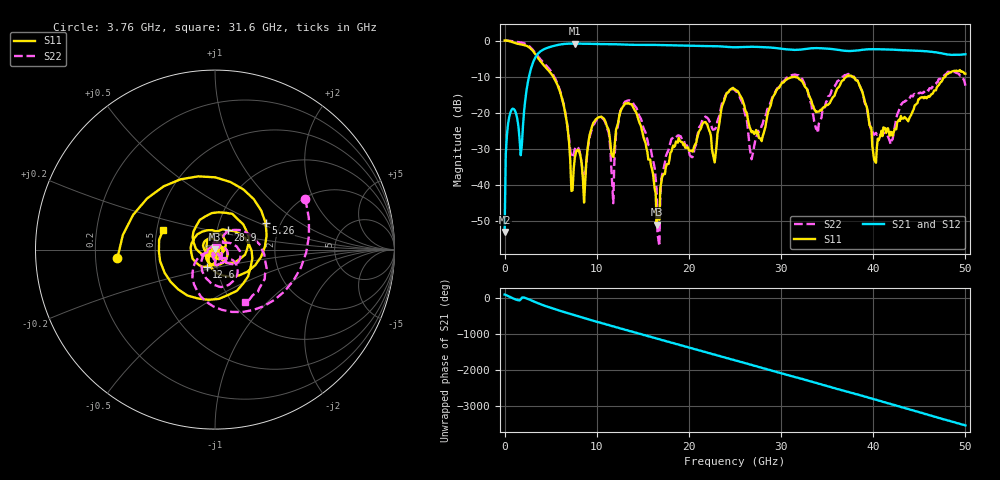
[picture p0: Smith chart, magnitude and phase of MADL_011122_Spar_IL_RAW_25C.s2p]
#	HZ	S	DB	R	50
!Frequency	S11 (dB)	S11-Ang	S21 (dB)	S21-Ang	S12 (dB)	S12-Ang	S22 (dB)	S22-Ang
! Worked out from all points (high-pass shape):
!   401 points, 10 MHz to 50 GHz, reference 50 ohm
!   highest |S21| = -0.85 dB at 7.63 GHz (marker M1); lowest = -53.1 dB at 10 MHz (marker M2)
!   |S21| within 3 dB of the highest: 3.567 GHz to 48 GHz (44.43 GHz wide, 172 % of centre); 49.825 GHz to end of sweep
!   lowest |S11| = -51.0 dB at 16.5 GHz (marker M3), VSWR 1.01, Z = 49.8 + j0.209 ohm
!   |S11| at or under -10 dB: 5.275 GHz to 37.1 GHz (31.83 GHz wide, 150 % of centre); 37.71 GHz to 47.82 GHz (10.1 GHz wide, 23.6 % of centre)
!   |S22| runs from -57.0 to 0.0 dB; largest |S21 - S12| = 0.016
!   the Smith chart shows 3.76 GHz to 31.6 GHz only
!   S11 on the Smith chart (normalised r, x): 3.76 GHz: 0.29, -0.04; 5.26 GHz: 1.67, +0.55; 12.6 GHz: 0.90, -0.17; 28.9 GHz: 1.12, +0.25; 31.6 GHz: 0.54, +0.13
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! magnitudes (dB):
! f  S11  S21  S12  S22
! 10 MHz  0.0  -53.1  -53.8  0.0
! 635 MHz  -0.3  -20.0  -20.0  -0.1
! 1.76 GHz  -1.1  -31.8  -31.7  -0.5
! 3.76 GHz  -5.3  -3.3  -3.3  -4.8
! 5.26 GHz  -9.9  -1.5  -1.5  -9.4
! 7.63 GHz  -32.4  -0.8  -0.8  -30.1
! 8.38 GHz  -34.2  -0.9  -0.9  -34.3
! 10.4 GHz  -21.2  -1.0  -1.0  -21.4
! 11.8 GHz  -32.3  -1.0  -1.0  -45.1
! 12.6 GHz  -19.5  -1.1  -1.1  -19.3
! 14.8 GHz  -23.7  -1.2  -1.2  -21.7
! 16.5 GHz  -51.0  -1.2  -1.2  -41.2
! 16.8 GHz  -49.7  -1.2  -1.2  -57.0
! 18.1 GHz  -30.8  -1.3  -1.3  -27.3
! 25.1 GHz  -13.8  -1.9  -1.8  -14.1
! 26.9 GHz  -25.1  -1.7  -1.7  -31.8
! 28.9 GHz  -17.8  -1.9  -1.9  -16.9
! 31.6 GHz  -10.2  -2.6  -2.6  -9.5
! 33.4 GHz  -17.8  -2.1  -2.1  -19.9
! 37.4 GHz  -9.8  -2.9  -2.9  -9.5
! 41.8 GHz  -26.4  -2.5  -2.5  -27.9
! 50 GHz  -9.2  -3.8  -3.8  -12.5
